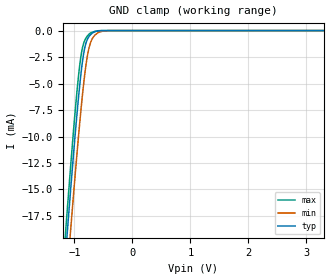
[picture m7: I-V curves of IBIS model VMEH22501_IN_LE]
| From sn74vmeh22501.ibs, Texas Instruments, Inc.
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[Model]   VMEH22501_IN_LE
Model_type  Input
Vinl=0.8V
Vinh=2.0V
| variable   typ   min   max
C_comp   2.53pF   1.97pF   3.21pF
[Temperature Range]   40   100   0
| Ambient temperature   25   85   0
[Voltage range]   3.3   3.15   3.45
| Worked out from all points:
|   GND clamp passes 1 mA (typ) near -0.79 V on its own axis
[GND Clamp]
| VMEH22501_IN_LE
|   Voltage   I(typ)   I(min)   I(max)
-5.5V     -362.8mA   -359.2mA   -369.8mA
-1.165V   -22.11mA   -25.83mA   -20.01mA
-1.135V   -19.96mA   -23.72mA   -17.82mA
-1.11V    -18.19mA   -21.98mA   -16.02mA
-1.085V   -16.45mA   -20.25mA   -14.25mA
-1.06V    -14.72mA   -18.53mA   -12.5mA
-950mV    -7.571mA   -11.3mA    -5.432mA
-875mV    -3.548mA   -6.849mA   -2.029mA
-820mV    -1.606mA   -4.085mA   -918.1uA
-755mV    -616.2uA   -1.814mA   -381.7uA
-625mV    -72.29uA   -327.4uA   -40.66uA
3.3V      21.02pA    116.2pA    16.36pA
